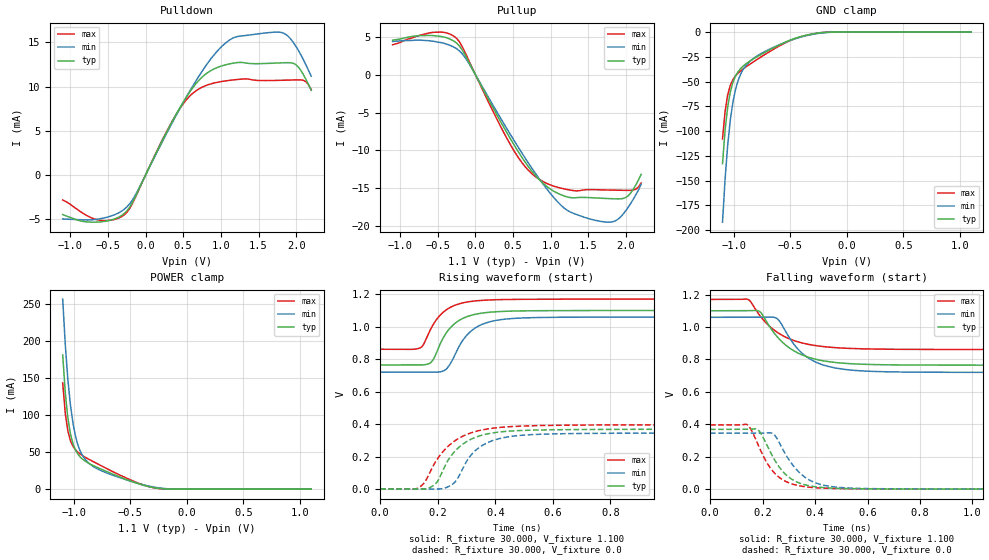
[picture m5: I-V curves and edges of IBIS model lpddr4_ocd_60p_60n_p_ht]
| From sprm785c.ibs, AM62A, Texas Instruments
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|   Model lpddr4_ocd_60p_60n_p_ht
[Model] lpddr4_ocd_60p_60n_p_ht
Model_type I/O
Polarity   Non-Inverting
Enable   Active-High
Vinl =  0.113V
Vinh =  0.253V
Vmeas =  0.183V
C_comp   2.659pF   2.613pF   2.734pF
C_comp_pullup   0.232pF   0.231pF   0.242pF
C_comp_pulldown   1.079pF   1.057pF   1.105pF
[Model Spec]
Vinh   0.253V   0.247V   0.265V
Vinl   0.113V   0.107V   0.125V
Vmeas   0.183V   0.176V   0.195V
[Temperature Range]   25.000   0.125k   -40.000
[Voltage Range]   1.100V   1.060V   1.170V
[Pullup Reference]   1.100V   1.060V   1.170V
[Pulldown Reference]   0.0V   0.0V   0.0V
[C Comp Corner]
C_comp_pullup   0.232pF   0.231pF   0.242pF
C_comp_pulldown   1.079pF   1.057pF   1.105pF
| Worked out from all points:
|   slope of the pulldown table from 0 to 0.165 V, typ, clamps not added: 56.7 ohm
|   slope of the pullup table from 0 to 0.165 V, typ, clamps not added: 53.1 ohm
|   GND clamp passes 1 mA (typ) near -0.26 V on its own axis
|   POWER clamp passes 1 mA (typ) near -0.24 V on its own axis
|   rising waveform, R_fixture 30.000, V_fixture 1.100: 20-80 % time 75.6ps typ, 81.1ps min, 74.4ps max; typ from 0.765 V to 1.1 V
|   rising waveform, R_fixture 30.000, V_fixture 0.0: 20-80 % time 95.6ps typ, 92.1ps min, 111ps max; typ from 0.001 V to 0.37 V
|   falling waveform, R_fixture 30.000, V_fixture 1.100: 20-80 % time 130ps typ, 116ps min, 135ps max; typ from 1.1 V to 0.765 V
|   falling waveform, R_fixture 30.000, V_fixture 0.0: 20-80 % time 90.8ps typ, 98.2ps min, 86.5ps max; typ from 0.369 V to 0.001 V
[Pulldown]
|Voltage   I(typ)   I(min)   I(max)
-1.1V     -4.465mA   -4.958mA   -2.813mA
-658mV    -5.322mA   -5.01mA    -5.016mA
-284mV    -4.35mA    -3.873mA   -4.5mA
-147mV    -2.645mA   -2.437mA   -2.741mA
261mV     4.542mA    4.396mA    4.609mA
533mV     8.695mA    8.688mA    8.416mA
805mV     11.45mA    12.41mA    10.13mA
1.145V    12.62mA    15.42mA    10.73mA
1.826V    12.69mA    16.06mA    10.72mA
2.03V     12.2mA     14.08mA    10.76mA
2.132V    10.78mA    12.41mA    10.53mA
2.2V      9.575mA    11.17mA    9.654mA
[Pullup]
|Voltage   I(typ)   I(min)   I(max)
-1.1V     4.549mA    4.382mA    3.953mA
-556mV    5.158mA    4.411mA    5.598mA
-249mV    4.161mA    3.422mA    4.791mA
-113mV    2.159mA    1.908mA    2.412mA
329mV     -6.101mA   -5.654mA   -6.734mA
601mV     -10.67mA   -10.08mA   -11.38mA
907mV     -14.41mA   -14.55mA   -14.16mA
1.247V    -16.2mA    -18.06mA   -15.21mA
1.622V    -16.28mA   -19.28mA   -15.18mA
1.86V     -16.38mA   -19.28mA   -15.24mA
2.03V     -15.96mA   -17.47mA   -15.26mA
2.2V      -13.15mA   -14.46mA   -14.29mA
[GND_clamp]
|Voltage   I(typ)   I(min)   I(max)
-1.1V     -132.9mA   -192.1mA   -107.9mA
-1.077V   -98.86mA   -148mA     -79.9mA
-1.054V   -75.63mA   -114.1mA   -63.35mA
-1.031V   -60.5mA    -88.93mA   -53.84mA
-1.008V   -50.81mA   -70.83mA   -48.11mA
-985mV    -44.46mA   -58.02mA   -44.3mA
-940mV    -36.83mA   -42.48mA   -39.19mA
-894mV    -32.12mA   -34.02mA   -35.3mA
-825mV    -26.95mA   -26.56mA   -29.98mA
-504mV    -8.258mA   -8.592mA   -8.733mA
-252mV    -912.8uA   -1.351mA   -908.2uA
1.1V      0A         0A         0A
[POWER_clamp]
|Voltage   I(typ)   I(min)   I(max)
-1.1V     181.7mA    257.3mA    143.9mA
-1.077V   130mA      195.2mA    102.2mA
-1.054V   95.89mA    147.8mA    78.5mA
-1.031V   74.31mA    112.9mA    65.32mA
-1.008V   60.91mA    88.11mA    57.78mA
-985mV    52.38mA    70.63mA    52.94mA
-940mV    42.73mA    49.84mA    46.89mA
-848mV    33.32mA    32.69mA    38.81mA
-710mV    23.85mA    21.95mA    27.87mA
-481mV    10mA       9.999mA    11.31mA
-252mV    1.151mA    1.835mA    969.3uA
1.1V      0A         0A         0A
[Ramp]
| variable   typ   min   max
dV/dt_r   0.224/66.061p   0.208/70.216p   0.245/67.594p
dV/dt_f   0.224/0.129n   0.208/0.126n   0.245/0.137n
R_load = 30.000
[Rising Waveform]
R_fixture= 30.000
V_fixture= 1.100
V_fixture_min= 1.060
V_fixture_max= 1.170
|time   V(typ)   V(min)   V(max)
0s        764.7mV    720.1mV    861.3mV
141ps     764.3mV    720.1mV    871.7mV
180ps     787.4mV    719.7mV    1V
220ps     934.5mV    728.1mV    1.09V
260ps     1.021V     828.1mV    1.132V
286ps     1.05V      913.3mV    1.146V
316ps     1.07V      973.5mV    1.156V
364ps     1.086V     1.021V     1.163V
433ps     1.095V     1.046V     1.167V
5ns       1.1V       1.06V      1.17V
[Rising Waveform]
R_fixture= 30.000
V_fixture= 0.0
V_fixture_min= 0.0
V_fixture_max= 0.0
|time   V(typ)   V(min)   V(max)
0s        839uV      1.261mV    1.781mV
135ps     800uV      1.26mV     10.87mV
157ps     1.959mV    1.259mV    50.07mV
192ps     33.27mV    1.294mV    168.1mV
231ps     163.6mV    11.85mV    256.1mV
279ps     266.6mV    99.03mV    319.3mV
309ps     302mV      195.7mV    343.2mV
344ps     327.7mV    257.1mV    361.4mV
480ps     361mV      330.4mV    387.8mV
5ns       369.5mV    346.7mV    396.5mV
[Falling Waveform]
R_fixture= 30.000
V_fixture= 1.100
V_fixture_min= 1.060
V_fixture_max= 1.170
|time   V(typ)   V(min)   V(max)
0s        1.1V       1.06V      1.17V
146ps     1.1V       1.06V      1.168V
191ps     1.093V     1.06V      1.067V
248ps     954.7mV    1.058V     976.1mV
266ps     921.5mV    1.033V     956.7mV
329ps     844.5mV    874.3mV    911.5mV
385ps     808.5mV    798.5mV    889.8mV
472ps     782.2mV    749mV      873.3mV
606ps     769.2mV    727.2mV    864.6mV
5ns       764.7mV    720.1mV    861.3mV
[Falling Waveform]
R_fixture= 30.000
V_fixture= 0.0
V_fixture_min= 0.0
V_fixture_max= 0.0
|time   V(typ)   V(min)   V(max)
0s        369.2mV    345.8mV    396.4mV
143ps     369.1mV    345.8mV    396.4mV
185ps     362.8mV    345.8mV    266.7mV
237ps     206.7mV    345mV      115.9mV
273ps     117.7mV    258.2mV    62.51mV
310ps     63.38mV    160.2mV    34.08mV
361ps     28.03mV    74.94mV    16.1mV
422ps     11.91mV    29.47mV    7.862mV
749ps     1.679mV    2.427mV    2.248mV
5ns       842.1uV    1.274mV    1.785mV
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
